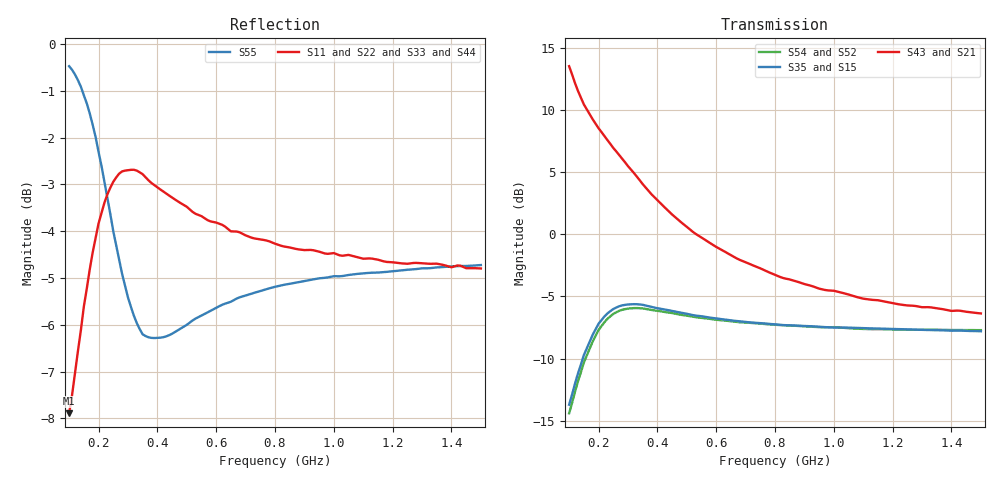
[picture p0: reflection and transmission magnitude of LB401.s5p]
!  POLYFET RF DEVICES
!  LB401 (Each Side)
!  S PARAMETERS
!  VDS=28V, IDQ=600mA
! Date: Wed Apr 07 15:05:08 1999
! SCATTERING PARAMETERS :
!AWR Design Environment (2053) Wed Feb 04 14:55:31 2004
!freq-unit  param-type  data-format  keyword  impedance-ohms
# MHz  S  MA  R  50
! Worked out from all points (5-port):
!   141 points, 100 MHz to 1.5 GHz, reference 50 ohm
!   strongest paths, dB at 100 MHz, 450 MHz, 800 MHz, 1.15 GHz, 1.5 GHz:
!     S43: 13.5, 1.6, -3.3, -5.3, -6.4
!     S21: 13.5, 1.6, -3.3, -5.3, -6.4
!     S35: -13.7, -6.2, -7.2, -7.6, -7.8
!     S15: -13.7, -6.2, -7.2, -7.6, -7.8
!     S54: -14.4, -6.3, -7.3, -7.6, -7.7
!     S52: -14.4, -6.3, -7.3, -7.6, -7.7
!   lowest |S11| = -7.9 dB at 100 MHz (marker M1), VSWR 2.35, Z = 40.4 - j38.4 ohm
!   |S11| at or under -10 dB: nowhere
